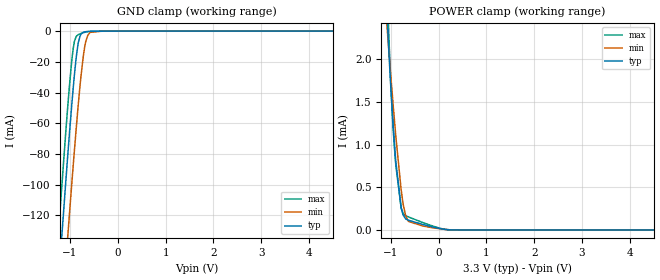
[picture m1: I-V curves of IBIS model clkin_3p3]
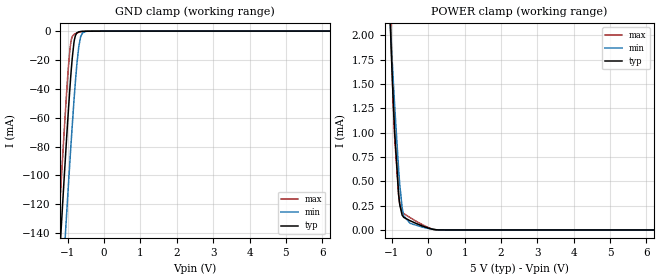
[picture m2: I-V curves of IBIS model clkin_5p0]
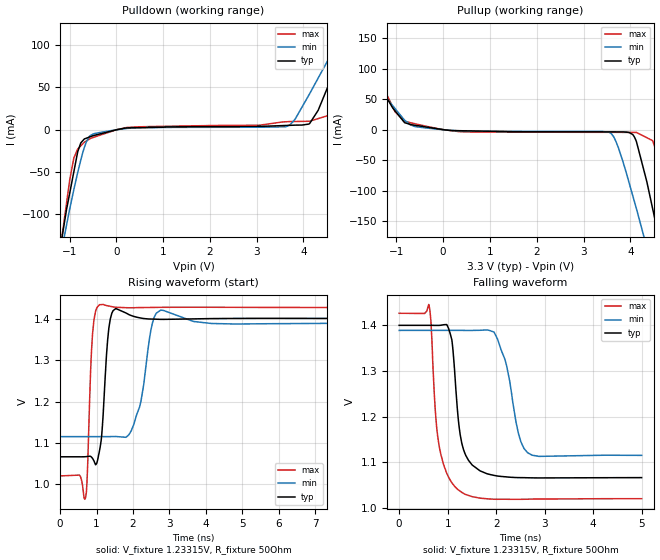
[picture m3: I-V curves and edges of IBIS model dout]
|Texas Instruments Incorporated
| AMC1305x 20-MHz, Isolated Delta-Sigma Modulator for Shunt-Based
| Current Measurement
| Marketing part#   Digital Voltage Range   Package-type   #pins
| AMC1305L25   2.7V-5.5V   SOIC   16
[IBIS Ver]   4.1
[File name]   amc1305l25.ibs
[File Rev]   1.1
[Date]   11/03/2014
[Source]
| Texas Instruments Incorporated.
| Analog-eLab Design Center, HPA
| 12500 TI Blvd
| Dallas, TX -75243
[Notes]   Revision History:
| Rev 1.1: 11/03/2014
| - Updated min corner voltage to 3V for 3.3V model.
| - Both p and n pad behaves symmetrically.Hence keeping only one model.
| Rev 1.0: 10/15/2014
| - Initial version of the model
| - Model generated from simulations in TISPICE
| - Model matched to SPICE simulation
| - C_comp although listed in numerical order of value are
|   obtained from varying PVT conditions. For PVT conditions for
|   each specific value refer the buffer description under
|   respective [Model]. IBIS model user is responsible for using
|   appropriate C_comp to simulate for Signal Integrity.
|* EXCEPTION:   *
|* -For model clkin_* there will be leakage current in  POWER clamp   *
|*  and GROUND clamp because of the the resistor(R0) connected to pad.   *
[Disclaimer]
| This model is designed as an aid for customers of Texas Instruments.
| TI and its licensors and suppliers make no warranties, either expressed
| or implied, with respect to this  model, including the warranties of
| merchantability or fitness for a particular purpose. The model is
| provided solely on an "as is" basis. The entire risk as to its quality
| and performance is with the customer.
[Copyright]
(C) Copyright 2014 Texas Instruments Incorporated.All rights reserved.
|   AMC1305L25
[Component]   AMC1305L25
[Manufacturer]   TI
[Package]   |16 SOIC
|   typ   min   max
R_pkg   0.2   0.16   0.24
L_pkg   1.5nH   1.2nH   1.8nH
C_pkg   0.4pF   0.32pF   0.48pF
[Pin]  signal_name   model_name   R_pin   L_pin   C_pin
1   NC   NC   NA   NA   NA
2   AINP   NC   NA   NA   NA
3   AINN   NC   NA   NA   NA
4   NC   NC   NA   NA   NA
5   NC   NC   NA   NA   NA
6   NC   NC   NA   NA   NA
7   AVDD   POWER   NA   NA   NA
8   AGND   GND   NA   NA   NA
9   DGND   GND   NA   NA   NA
10   DOUT_N   dout   NA   NA   NA
11   DOUT   dout   NA   NA   NA
12   CLKIN_N   CLKIN   NA   NA   NA
13   CLKIN   CLKIN   NA   NA   NA
14   DVDD   POWER   NA   NA   NA
15   NC   NC   NA   NA   NA
16   DGND   GND   NA   NA   NA
[Diff_pin]   inv_pin   vdiff   tdelay_typ   tdelay_min   tdelay_max
11   10   NA   NA   NA   NA
13   12   0.2   NA   NA   NA
|   Model Selectors
[Model Selector] CLKIN
clkin_3p3   3.3V   Differential input
clkin_5p0   5.0V   Differential input
| Models and submodels in the file (3): clkin_3p3 (Input), clkin_5p0 (Input), dout (Output)
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|   clkin_3p3 Model
[Model]   clkin_3p3
Model_type   Input
Vinl = 0.99
Vinh = 2.31
|   typ   min   max
|   (nom PVT)   (fast PVT)   (slow PVT)
C_comp   3.817e-13   3.282e-13   4.211e-13
| Where nom  PVT is Nominal Process, 3.3V, 27C
|   Fast PVT is Strong Process,  3.6V, -40C
|   Slow PVT is Weak Process,   3.0V, 125C
[Model spec]
|subparameter
Vinl   0.99   0.90   1.08
Vinh   2.31   2.10   2.52
[Voltage Range]   3.3   3   3.6
|Junction Temperature
[Temperature Range]   27   125   -40
[Power Clamp Reference]   3.3   3   3.6
[GND Clamp Reference]   0   0   0
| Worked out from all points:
|   GND clamp passes 1 mA (typ) near -0.73 V on its own axis
|   POWER clamp passes 1 mA (typ) near -0.92 V on its own axis
[GND Clamp]
|   Voltage   I(typ)   I(min)   I(max)
-3.3V     -1.107A    -1.149A    -1.083A
-1.545V   -299mA     -350.2mA   -268.4mA
-1.194V   -143mA     -195.9mA   -110.5mA
-1.09V    -98.49mA   -151.5mA   -66.14mA
-1.038V   -77.24mA   -129.9mA   -45.48mA
-934.8mV  -37.68mA   -88.12mA   -11.74mA
-873.6mV  -18.18mA   -64.63mA   -3.708mA
-825mV    -7.38mA    -47.11mA   -2.297mA
-720mV    -760.3uA   -15.89mA   -1.027mA
-630mV    -236.9uA   -2.827mA   -400.2uA
-330mV    -71.67uA   -52.11uA   -95.33uA
6.6V      0A         0A         0A
[POWER Clamp]
|   Voltage   I(typ)   I(min)   I(max)
-3.3V     31.3mA     24.87mA    37.98mA
-1.075V   2.46mA     2.344mA    2.762mA
-1.033V   1.992mA    2.03mA     2.138mA
-999.6mV  1.656mA    1.791mA    1.692mA
-956.4mV  1.263mA    1.492mA    1.213mA
-897.6mV  805.5uA    1.104mA    762.7uA
-783.6mV  256.1uA    463.8uA    256.1uA
-742.5mV  172.6uA    299uA      192uA
-689.7mV  129.7uA    163.8uA    166.8uA
-633mV    114uA      100.3uA    152.7uA
231.6mV   1.663uA    2.329uA    1.816uA
6.6V      0A         0A         0A
|   clkin_5p0 Model
[Model]   clkin_5p0
Model_type   Input
Vinl = 1.5
Vinh = 3.5
|   typ   min   max
|   (nom PVT)   (fast PVT)   (slow PVT)
C_comp   3.559e-13   3.082e-13   3.874e-13
| Where nom  PVT is Nominal Process, 5V, 27C
|   Fast PVT is Strong Process,  5.5V, -40C
|   Slow PVT is Weak Process,   4.5V, 125C
[Model spec]
|subparameter
Vinl   1.5   1.35   1.65
Vinh   3.5   3.15   3.85
[Voltage Range]   5   4.5   5.5
|Junction Temperature
[Temperature Range]   27   125   -40
[Power Clamp Reference]   5   4.5   5.5
[GND Clamp Reference]   0   0   0
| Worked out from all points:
|   GND clamp passes 1 mA (typ) near -0.73 V on its own axis
|   POWER clamp passes 1 mA (typ) near -0.92 V on its own axis
[GND Clamp]
|   Voltage   I(typ)   I(min)   I(max)
-5V       -1.894A    -1.931A    -1.874A
-1.26V    -171.8mA   -224.5mA   -139.6mA
-1.175V   -134.8mA   -187.8mA   -102.3mA
-1.1V     -102.8mA   -155.8mA   -70.44mA
-1.034V   -75.82mA   -128.5mA   -44.13mA
-941mV    -39.88mA   -90.56mA   -13.2mA
-900.5mV  -26.16mA   -74.79mA   -5.88mA
-825.5mV  -7.466mA   -47.29mA   -2.307mA
-698mV    -547.7uA   -11.27mA   -836.8uA
-594.5mV  -173.3uA   -1.218mA   -273uA
-462.5mV  -99.15uA   -104.2uA   -131.4uA
10V       0A         0A         0A
[POWER Clamp]
|   Voltage   I(typ)   I(min)   I(max)
-5V       49.42mA    39.69mA    59.34mA
-1.046V   2.128mA    2.123mA    2.32mA
-1.012V   1.784mA    1.883mA    1.861mA
-968mV    1.365mA    1.572mA    1.333mA
-924.5mV  1.005mA    1.279mA    949.9uA
-814.5mV  361.9uA    617.6uA    357.8uA
-781.5mV  256uA      456.2uA    257.1uA
-720mV    153.3uA    233.5uA    183.2uA
-675.5mV  129.5uA    145uA      168.1uA
-500mV    94.82uA    69.02uA    126.8uA
255mV     1.034uA    1.351uA    1.6uA
10V       0A         0A         0A
|   dout Model
[Model]   dout
Model_type   Output
Polarity   Non-Inverting
Vmeas = 1.2
Vref = 1.23
Cref = 5pF
Rref = 50
|   typ   min   max
|   (nom PVT)   (fast PVT)   (slow PVT)
C_comp   1.893e-12   1.832e-12   2.035e-12
| Where nom  PVT is Nominal Process, 3.3V, 27C
|   Fast PVT is Strong Process,  3.6V, -40C
|   Slow PVT is Weak Process,   3.0V, 125C
[Voltage Range]   3.3   3.0   3.6
|Junction Temperature
[Temperature Range]   27   125   -40
[Pullup Reference]   3.3   3.0   3.6
[Pulldown Reference]   0   0   0
[Power Clamp Reference]   3.3   3.0   3.6
[GND Clamp Reference]   0   0   0
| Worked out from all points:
|   slope of the pulldown table from 0 to 0.495 V, typ, clamps not added: 195 ohm
|   slope of the pullup table from 0 to 0.495 V, typ, clamps not added: 257 ohm
|   falling waveform, V_fixture 1.23315V, R_fixture 50Ohm: 20-80 % time 194ps typ, 298ps min, 216ps max; typ from 1.4 V to 1.07 V
|   rising waveform, V_fixture 1.23315V, R_fixture 50Ohm: 20-80 % time 137ps typ, 316ps min, 102ps max; typ from 1.07 V to 1.4 V
[Pulldown]
|   Voltage   I(typ)   I(min)   I(max)
-3.3V     -917.4mA   -770.8mA   -1.099A
-1.414V   -214.3mA   -211.6mA   -228.4mA
-1.066V   -95.1mA    -113.5mA   -87.83mA
-906mV    -49.33mA   -70.41mA   -33.13mA
-642mV    -10.04mA   -14.55mA   -13.39mA
-2.4mV    -118.2uA   -88.42uA   -144.1uA
3.627V    5.043mA    3.61mA     9.439mA
4.132V    7.347mA    42.63mA    10.08mA
4.588V    59.88mA    88.85mA    17.82mA
4.983V    113.2mA    126.2mA    80.51mA
5.286V    147.2mA    150.1mA    133.2mA
6.6V      249.6mA    222.9mA    273.6mA
[Pullup]
|   Voltage   I(typ)   I(min)   I(max)
-3.3V     249.8mA    209.3mA    295.1mA
-2.17V    167.5mA    141.5mA    199.1mA
-1.774V   124.6mA    104.7mA    147.4mA
-1.025V   30.63mA    34.37mA    28.95mA
-603mV    7.3mA      5.189mA    9.82mA
3.555V    -3.495mA   -4.355mA   -4.232mA
4.13V     -19.73mA   -129.5mA   -4.394mA
4.476V    -129.1mA   -228.1mA   -17.93mA
4.663V    -195.8mA   -283.1mA   -73.89mA
4.828V    -254.4mA   -331.4mA   -146.4mA
5.022V    -327mA     -388.4mA   -232mA
6.6V      -917.2mA   -861.1mA   -958.5mA
[Ramp]
R_load = 50
|   typ   min   max
dV/dt_r   0.100337/8.6013e-11   0.0821544/1.22758e-10  0.122323/7.74057e-11
dV/dt_f   0.200052/1.92471e-10  0.164171/2.96524e-10   0.243555/2.14279e-10
[Falling Waveform]
V_fixture = 1.23315V
V_fixture_min = 1.25219V
V_fixture_max = 1.22316V
R_fixture = 50Ohm
|   Time   V(typ)   V(min)   V(max)
0s        1.4V       1.389V     1.426V
614ps     1.4V       1.389V     1.445V
746ps     1.4V       1.389V     1.212V
826ps     1.4V       1.389V     1.135V
1.086ns   1.368V     1.389V     1.055V
1.222ns   1.192V     1.389V     1.039V
1.43ns    1.104V     1.389V     1.028V
1.96ns    1.071V     1.384V     1.019V
2.65ns    1.066V     1.121V     1.019V
5ns       1.067V     1.115V     1.02V
[Rising Waveform]
V_fixture = 1.23315V
V_fixture_min = 1.25219V
V_fixture_max = 1.22316V
R_fixture = 50Ohm
|   Time   V(typ)   V(min)   V(max)
0s        1.067V     1.115V     1.02V
696ps     1.067V     1.115V     967.2mV
886ps     1.063V     1.115V     1.359V
1.086ns   1.084V     1.115V     1.434V
1.334ns   1.375V     1.115V     1.43V
1.524ns   1.424V     1.116V     1.427V
2.018ns   1.405V     1.144V     1.426V
2.536ns   1.399V     1.39V      1.427V
2.756ns   1.398V     1.42V      1.427V
10ns      1.4V       1.389V     1.426V
